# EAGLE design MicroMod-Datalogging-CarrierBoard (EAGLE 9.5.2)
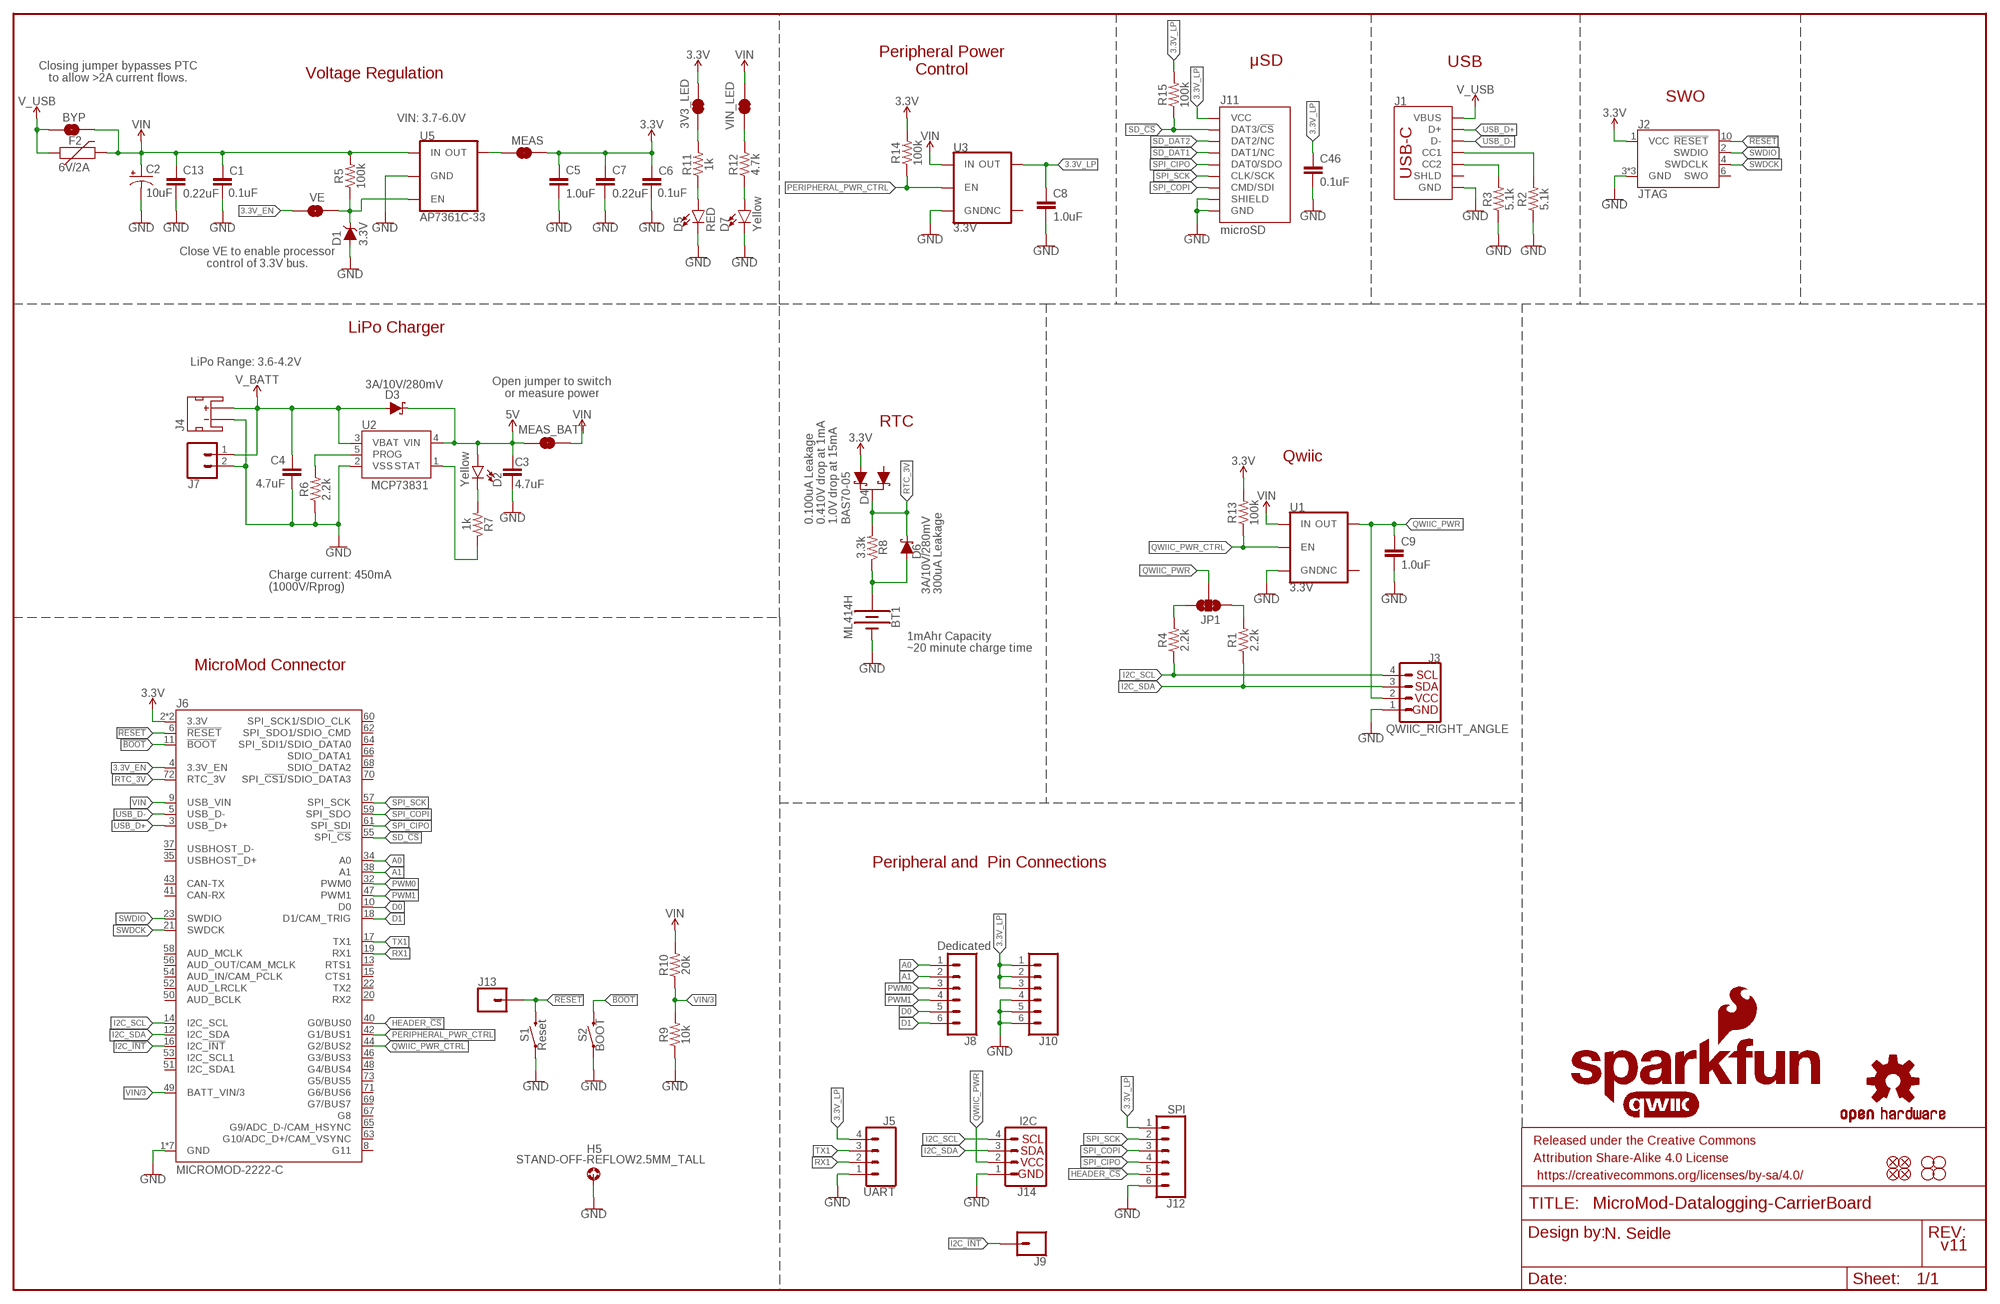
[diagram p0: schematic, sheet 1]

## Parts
3V3_LED  JUMPER-SMT_2_NC_TRACE_SILK  [SMT-JUMPER_2_NC_TRACE_SILK]
BT1  ML414H  ML414H_IV01E_BATTERY  [ML414H_IV01E]
BYP  JUMPER-SMT_2_NO_SILK  [SMT-JUMPER_2_NO_SILK]
C1  0.1uF  0.1UF-0603-25V-(+80/-20%)  [0603]
C2  10uF  10UF-POLAR-EIA3216-16V-10%(TANT)  [EIA3216]
C3  4.7uF  4.7UF-0603-35V-(20%)  [0603]
C4  4.7uF  4.7UF-0603-6.3V-(10%)  [0603]
C5  1.0uF  1.0UF-0603-16V-10%  [0603]
C6  0.1uF  0.1UF-0603-25V-(+80/-20%)  [0603]
C7  0.22uF  0.22UF-0603-25V-10%  [0603]
C8  1.0uF  1.0UF-0603-16V-10%  [0603]
C9  1.0uF  1.0UF-0603-16V-10%  [0603]
C13  0.22uF  0.22UF-0603-25V-10%  [0603]
C46  0.1uF  0.1UF-0603-25V-(+80/-20%)  [0603]
D1  3.3V  DIODE-ZENER-MM3Z3V3T1G  [SOD-323]
D2  Yellow  LED-YELLOW0603  [LED-0603]
D3  3A/10V/280mV  DIODE-SCHOTTKY-BAT60A  [SOD-323]
D4  BAS70-05  DIODE-SCHOTTKY-DUAL  [SOT23-3]
D5  RED  LED-RED0603  [LED-0603]
D6  3A/10V/280mV  DIODE-SCHOTTKY-BAT60A  [SOD-323]
D7  Yellow  LED-YELLOW0603  [LED-0603]
F2  6V/2A  PPTC_6V2A  [1210]
FD1  FIDUCIALUFIDUCIAL  [FIDUCIAL-MICRO]
FD2  FIDUCIALUFIDUCIAL  [FIDUCIAL-MICRO]
FD3  FIDUCIALUFIDUCIAL  [FIDUCIAL-MICRO]
FD4  FIDUCIALUFIDUCIAL  [FIDUCIAL-MICRO]
FRAME1  FRAME-LEDGER  [CREATIVE_COMMONS]
H1  STAND-OFF  [STAND-OFF]
H2  STAND-OFF  [STAND-OFF]
H3  STAND-OFF  [STAND-OFF]
H4  STAND-OFF  [STAND-OFF]
H5  STAND-OFF-REFLOW2.5MM_TALL  [STAND-OFF-REFLOW-M2.5]
J1  USB_C_2-LAYER_PADS  [USB-C-16P-2LAYER-PADS]
J2  JTAG  CORTEX_JTAG_DEBUG_MINIMUM_PTH  [2X5-PTH-1.27MM]
J3  QWIIC_RIGHT_ANGLE  QWIIC_CONNECTORJS-1MM  [JST04_1MM_RA]
J4  JST_2MM_MALE  [JST-2-SMD]
J5  UART  CONN_041X04_NO_SILK  [1X04_NO_SILK]
J6  MICROMOD-2222-C  [M.2-CONNECTOR-E]
J7  CONN_021X02_NO_SILK  [1X02_NO_SILK]
J8  Dedicated  CONN_06NO_SILK_NO_POP  [1X06_NO_SILK]
J9  CONN_01PTH_NO_SILK_YES_STOP  [1X01_NO_SILK]
J10  CONN_06NO_SILK_NO_POP  [1X06_NO_SILK]
J11  microSD  MICRO-SD-SDIOPUSH-PUSH  [MICRO-SD-SOCKET]
J12  SPI  CONN_06NO_SILK_NO_POP  [1X06_NO_SILK]
J13  CONN_01PTH_NO_SILK_YES_STOP  [1X01_NO_SILK]
J14  I2C  I2C_STANDARD_NO_SILK  [1X04_NO_SILK]
JP1  JUMPER-SMT_3_2-NC_TRACE_SILK  [SMT-JUMPER_3_2-NC_TRACE_SILK]
LOGO1  SFE_LOGO_NAME_FLAME.1_INCH  [SFE_LOGO_NAME_FLAME_.1]
LOGO2  QWIIC_LOGO_CONNECTOR  [QWIIC_5.5MM]
LOGO3  OSHW-LOGOMINI  [OSHW-LOGO-MINI]
MEAS  JUMPER-COMBO_2_NC_TRACE  [COMBO-JUMPER_2_NC_TRACE]
MEAS_BATT  JUMPER-COMBO_2_NC_TRACE  [COMBO-JUMPER_2_NC_TRACE]
R1  2.2k  2.2KOHM-0603-1/10W-1%  [0603]
R2  5.1k  5.1KOHM5.1KOHM-0603-1/10W-1%  [0603]
R3  5.1k  5.1KOHM5.1KOHM-0603-1/10W-1%  [0603]
R4  2.2k  2.2KOHM-0603-1/10W-1%  [0603]
R5  100k  100KOHM-0603-1/10W-1%  [0603]
R6  2.2k  2.2KOHM-0603-1/10W-1%  [0603]
R7  1k  1KOHM-0603-1/10W-1%  [0603]
R8  3.3k  3.3KOHM-0603-1/10W-1%  [0603]
R9  10k  10KOHM-0603-1/10W-1%  [0603]
R10  20k  20KOHM-0603-1/10W-1%  [0603]
R11  1k  1KOHM-0603-1/10W-1%  [0603]
R12  4.7k  4.7KOHM-0603-1/10W-1%  [0603]
R13  100k  100KOHM-0603-1/10W-1%  [0603]
R14  100k  100KOHM-0603-1/10W-1%  [0603]
R15  100k  100KOHM-0603-1/10W-1%  [0603]
S1  Reset  MOMENTARY-SWITCH-SPST-SMD-5.2-TALL-REDUNDANT  [TACTILE_SWITCH_SMD_5.2MM]
S2  BOOT  MOMENTARY-SWITCH-SPST-SMD-5.2-TALL-REDUNDANT  [TACTILE_SWITCH_SMD_5.2MM]
U1  3.3V  V_REG_AP2112K-3.3V  [SOT23-5]
U2  MCP73831  [SOT23-5]
U3  3.3V  V_REG_AP2112K-3.3V  [SOT23-5]
U5  AP7361C-33  AP7361C-33FGEUDFN-8  [UDFN-8]
VE  JUMPER-SMT_2_NO_SILK  [SMT-JUMPER_2_NO_SILK]
VIN_LED  JUMPER-SMT_2_NC_TRACE_SILK  [SMT-JUMPER_2_NC_TRACE_SILK]

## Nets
3.3V: 3V3_LED.2 C5.1 C6.1 C7.1 D4.2(A1) J2.1(VCC) J6.2(3.3V) J6.74(3.3V) MEAS.2 MEAS.4 R13.2 R14.2
3.3V_EN: J6.4(3.3V_EN) VE.1
3.3V_EN_VE: D1.C R5.1 U5.5(EN) VE.2
3.3V_LP: C8.1 C46.1 J5.4 J10.1 J10.2 J10.3 J11.VCC J12.1 R15.2 U3.5(OUT)
5V: C3.1 D2.A D3.C MEAS_BATT.1 MEAS_BATT.3 U2.4(VIN)
!BOOT!: J6.11(!BOOT!) S2.3 S2.4
!RESET!: J2.10(!RESET) J6.6(!RESET!) J13.1 S1.3 S1.4
A0: J6.34(A0) J8.1
A1: J6.38(A1) J8.2
CHG_LED: R7.1 U2.1(STAT)
D0: J6.10(D0) J8.5
D1: J6.18(D1/CAM_TRIG) J8.6
GND: BT1.- C1.2 C2.- C3.2 C4.2 C5.2 C6.2 C7.2 C8.2 C9.2 C13.2 C46.2 D1.A D5.C D7.C H5.1 J1.GND J1.GND2(GND) J2.3(GND) J2.5(GND) J2.9(GND) J3.1 J4.1(-) J5.1 J6.1(GND) J6.7(GND) J6.33(GND) J6.36(GND) J6.39(GND) J6.45(GND) J6.75(GND) J7.2 J10.4 J10.5 J10.6 J11.CD1(SHIELD) J11.GND J11.GND1(GND) J11.GND3(GND) J12.6 J14.1 R2.1 R3.1 R6.1 R9.1 S1.1 S1.2 S2.1 S2.2 U1.2(GND) U2.2(VSS) U3.2(GND) U5.4(GND) U5.EP(GND)
HEADER_!CS!: J6.40(G0/BUS0) J12.5
I2C_!INT!: J6.16(I2C_!INT!) J9.1
I2C_SCL: J3.4 J6.14(I2C_SCL) J14.4 R4.1
I2C_SDA: J3.3 J6.12(I2C_SDA) J14.3 R1.1
N$1: MEAS.1 MEAS.3 U5.1(OUT)
N$2: JP1.3 R4.2
N$3: JP1.1 R1.2
N$4: D2.C R7.2
N$5: D5.A R11.1
N$6: 3V3_LED.1 R11.2
N$7: R6.2 U2.5(PROG)
N$8: R12.2 VIN_LED.1
N$9: D7.A R12.1
N$10: J1.A5(CC1) R2.2
N$11: J1.B5(CC2) R3.2
N$14: BT1.+ D6.A R8.1
PERIPHERAL_PWR_CTRL: J6.42(G1/BUS1) R14.1 U3.3(EN)
PWM0: J6.32(PWM0) J8.3
PWM1: J6.47(PWM1) J8.4
QWIIC_PWR: C9.1 J3.2 J14.2 JP1.2 U1.5(OUT)
QWIIC_PWR_CTRL: J6.44(G2/BUS2) R13.1 U1.3(EN)
RTC_3V: D4.3(C) D6.C J6.72(RTC_3V) R8.2
RX1: J5.2 J6.19(RX1)
SD_!CS!: J6.55(SPI_!CS!) J11.CS/DAT3(DAT3/!CS!) R15.1
SD_DAT1: J11.DAT1(DAT1/NC)
SD_DAT2: J11.DAT2(DAT2/NC)
SPI_CIPO: J6.61(SPI_SDI) J11.DO/DAT0(DAT0/SDO) J12.4
SPI_COPI: J6.59(SPI_SDO) J11.DI/CMD(CMD/SDI) J12.3
SPI_SCK: J6.57(SPI_SCK) J11.SCLK(CLK/SCK) J12.2
SWDCK: J2.4(SWDCLK) J6.21(SWDCK)
SWDIO: J2.2(SWDIO) J6.23(SWDIO)
TX1: J5.3 J6.17(TX1)
USB_D+: J1.A6(D+) J1.B6(D+) J6.3(USB_D+)
USB_D-: J1.A7(D-) J1.B7(D-) J6.5(USB_D-)
V_BATT: C4.1 D3.A J4.2(+) J7.1 U2.3(VBAT)
V_USB: BYP.1 F2.1 J1.VBUS1(VBUS) J1.VBUS2(VBUS)
VIN: BYP.2 C1.1 C2.+ C13.1 F2.2 J6.9(USB_VIN) MEAS_BATT.2 MEAS_BATT.4 R5.2 R10.2 U1.1(IN) U3.1(IN) U5.8(IN) VIN_LED.2
VIN/3: J6.49(BATT_VIN/3) R9.2 R10.1
Unconnected: D4.1(A) J1.SHLD1(SHLD) J1.SHLD2(SHLD) J1.SHLD3(SHLD) J1.SHLD4(SHLD) J2.6(SWO) J4.NC1(PAD1) J4.NC2(PAD2) J6.8(G11) J6.13(RTS1) J6.15(CTS1) J6.20(RX2) J6.22(TX2) J6.35(USBHOST_D+) J6.37(USBHOST_D-) J6.41(CAN-RX) J6.43(CAN-TX) J6.46(G3/BUS3) J6.48(G4/BUS4) J6.50(AUD_BCLK) J6.51(I2C_SDA1) J6.52(AUD_LRCLK) J6.53(I2C_SCL1) J6.54(AUD_IN/CAM_PCLK) J6.56(AUD_OUT/CAM_MCLK) J6.58(AUD_MCLK) J6.60(SPI_SCK1/SDIO_CLK) J6.62(SPI_SDO1/SDIO_CMD) J6.63(G10/ADC_D+/CAM_VSYNC) J6.64(SPI_SDI1/SDIO_DATA0) J6.65(G9/ADC_D-/CAM_HSYNC) J6.66(SDIO_DATA1) J6.67(G8) J6.68(SDIO_DATA2) J6.69(G7/BUS7) J6.70(SPI_!CS1!/SDIO_DATA3) J6.71(G6/BUS6) J6.73(G5/BUS5) U1.4(NC) U3.4(NC)

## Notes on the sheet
- Peripheral Power
  Control
- μSD | USB
- Closing jumper bypasses PTC
  to allow >2A current flows.
- Voltage Regulation
- SWO
- VIN: 3.7-6.0V
- Close VE to enable processor
  control of 3.3V bus.
- LiPo Charger
- LiPo Range: 3.6-4.2V
- Open jumper to switch
  or measure power
- RTC
- Qwiic
- 0.100uA Leakage
  0.410V drop at 1mA
  1.0V drop at 15mA
- Charge current: 450mA
  (1000V/Rprog)
- 300uA Leakage
- 1mAhr Capacity
- ~20 minute charge time
- MicroMod Connector
- Peripheral and  Pin Connections
- N. Seidle
- v11

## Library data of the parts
3V3_LED VIN_LED = SparkFun-Jumpers:JUMPER-SMT_2_NC_TRACE: Normally closed trace jumper
BT1 = SparkFun-Batteries:ML414H_IV01E_BATTERY: SEIKO ML414H-IV01E Reflowable Lithium Battery; PROD_ID: BATT-14267
BYP VE = SparkFun-Jumpers:JUMPER-SMT_2_NO: Normally open jumper
C1 C6 C46 = SparkFun-Capacitors:0.1UF: 0.1µF ceramic capacitors; PROD_ID: CAP-00810
C2 = SparkFun-Capacitors:10UF-POLAR: 10.0µF polarized capacitors; PROD_ID: CAP-00811
C3 = SparkFun-Capacitors:4.7UF: 4.7µF ceramic capacitors; PROD_ID: CAP-14106
C4 = SparkFun-Capacitors:4.7UF: 4.7µF ceramic capacitors; PROD_ID: CAP-08280
C5 C8 C9 = SparkFun-Capacitors:1.0UF: 1µF ceramic capacitors; PROD_ID: CAP-00868
C7 C13 = SparkFun-Capacitors:0.22UF: 0.22µF ceramic capacitors; PROD_ID: CAP-07822
D1 = SparkFun-DiscreteSemi:DIODE-ZENER: Zener Diode; PROD_ID: DIO-11284
D2 D7 = SparkFun-LED:LED-YELLOW: Yellow SMD LED; PROD_ID: DIO-09003
D3 D6 = SparkFun-DiscreteSemi:DIODE-SCHOTTKY: Schottky diode; PROD_ID: DIO-14072
D4 = SparkFun-DiscreteSemi:DIODE-SCHOTTKY-DUAL: Diodes Incorporated - BAS70-05 Dual Schottky Diode Two Schottky Diodes in a single SOT-23 package. Low reverse current (100 nA) Vf: Datasheet referenced for footprint; PROD_ID: DIO-14829
D5 = SparkFun-LED:LED-RED: Red SMD LED; PROD_ID: DIO-00819
F2 = SparkFun-Fuses:PPTC: Resettable Fuse PPTC; PROD_ID: RES-14313
FD1-FD4 = SparkFun-Aesthetics:FIDUCIAL: Fiducial Alignment Points
FRAME1 = SparkFun-Aesthetics:FRAME-LEDGER: Schematic Frame - Ledger
H1-H4 = SparkFun-Hardware:STAND-OFF: Stand Off
H5 = SparkFun-Hardware:STAND-OFF-REFLOW: Stand Off Reflow Compatible; PROD_ID: HW-14899
J1 = SparkFun-Connectors:USB_C: USB Type C 16Pin Connector Super Speed pins not available on the 16-pin purely SMD connector so this part is best for USB 2.0 implementations. D1 and D2 are tied together enabling D+/- no matter which way the cable is plugged into the connector. The two channel configuration pins (CC1/2) are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; PROD_ID: CONN-14122
J2 = SparkFun-Connectors:CORTEX_JTAG_DEBUG_MINIMUM: Cortex Debug Connector - 10 pin Supports JTAG debug, Serial Wire debug, and Serial Wire Viewer. PTH and SMD connector options available. General Connector Information Products: PTH Connector -via Digi-Key SparkFun PSoc SparkFun T
J3 = SparkFun-Connectors:QWIIC_CONNECTOR: SparkFun I2C Standard Qwiic Connector An SMD 1mm pitch JST connector makes it easy and quick (get it? Qwiic?) to connect I2C devices to each other. The Qwiic system enables fast and solderless connection between popular platforms and various sensors and actuators. We carry 200mm, 100mm, 50mm, and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; PROD_ID: CONN-13694
J4 = SparkFun-Connectors:JST_2MM_MALE: JST 2MM MALE RA CONNECTOR Two pin, compact surface mount connector. Commonly used as a battery input connection point. We really like the solid locking feeling and high current rating on these small connectors. We use these all the time as battery connectors. Mates to single-cell LiPo batteries.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; PROD_ID: CONN-11443; SF_ID: PRT-08612
J5 = SparkFun-Connectors:CONN_04: Multi connection point. Often used as Generic Header-pin footprint for 0.1 inch spaced/style header connections On any of the 0.1 inch spaced packages, you can populate with these: Break Away Headers - Straight (PRT-00116) Break Away Male Headers - Right Angle (PRT-00553) Female Headers (PRT-00115)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; PROD_ID: CONN-09696
J6 = SparkFun-MicroMod:MICROMOD: MicroMod Connector Description: A card edge connector and mating PCB connector to allow various MicroMod Processor Boards to be coupled with various carrier boards of different capabilities. Based on the M.2 standard.; PROD_ID: CONN-14877
J7 = SparkFun-Connectors:CONN_02: Multi connection point. Often used as Generic Header-pin footprint for 0.1 inch spaced/style header connections
J8 J10 J12 = SparkFun-Connectors:CONN_06: Multi connection point. Often used as Generic Header-pin footprint for 0.1 inch spaced/style header connections On any of the 0.1 inch spaced packages, you can populate with these: Break Away Headers - Straight (PRT-00116) Break Away Male Headers - Right Angle (PRT-00553) Female Headers (PRT-00115)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
J9 J13 = SparkFun-Connectors:CONN_01: Single connection point. Often used as Generic Header-pin footprint for 0.1 inch spaced/style header connections
J11 = SparkFun-Connectors:MICRO-SD-SDIO: microSD Socket for Transflash Push-push type µSD socket. tDoc lines correctly indicate media card edge positions when inserting (unlocked, locked, depressed). NOTE: CD1 and CD2 are connected internally, and the default detect state of the socket is detect pin to ground. SparkFun Products: WAV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; PROD_ID: CONN-07820
J14 = SparkFun-Connectors:I2C_STANDARD: SparkFun I2C Standard Pinout Header SparkFun has standardized on a pinout for all I2C based sensor breakouts. This pinout allows I2C boards to be plugged directly into the headers on Arduino Uno compatible boards, and to be daisy chained easily. Example SparkFun Products: SparkFun Atmospheric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
JP1 = SparkFun-Jumpers:JUMPER-SMT_3_2-NC_TRACE: Normally closed trace jumper (2 of 2 connections) This jumper has a trace between all three pads so they are normally closed (NC). Use a razor knife to open the connection(s). For best results follow the IPC guidelines for cutting traces: Cutout at least 0.063 mm (0.005 in). Remove all loose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
LOGO1 = SparkFun-Aesthetics:SFE_LOGO_NAME_FLAME: SparkFun Font Logo w/ Flame
LOGO2 = SparkFun-Aesthetics:QWIIC_LOGO: Qwiic Logos for placement on schematic and PCB. The 5.5mm silk logo is best for placing next to Qwiic connector.
LOGO3 = SparkFun-Aesthetics:OSHW-LOGO: Open-Source Hardware (OSHW) Logo
MEAS MEAS_BATT = SparkFun-Jumpers:JUMPER-COMBO_2_NC_TRACE
R1 R4 R6 = SparkFun-Resistors:2.2KOHM: 2.2kΩ resistor; PROD_ID: RES-08272
R2 R3 = SparkFun-Resistors:5.1KOHM; PROD_ID: RES-12083
R5 R13-R15 = SparkFun-Resistors:100KOHM: 100kΩ resistor; PROD_ID: RES-07828
R7 R11 = SparkFun-Resistors:1KOHM: 1kΩ resistor; PROD_ID: RES-07856
R8 = SparkFun-Resistors:3.3KOHM: 3.3kΩ resistor; PROD_ID: RES-07851
R9 = SparkFun-Resistors:10KOHM: 10kΩ resistor; PROD_ID: RES-00824
R10 = SparkFun-Resistors:20KOHM: 20kΩ resistor; PROD_ID: RES-09383
R12 = SparkFun-Resistors:4.7KOHM: 4.7kΩ resistor; PROD_ID: RES-07857
S1 S2 = SparkFun-Switches:MOMENTARY-SWITCH-SPST: Momentary Switch (Pushbutton) - SPST; PROD_ID: SWCH-14139
U1 U3 = SparkFun-IC-Power:V_REG_AP2112: AP2112 - 600mA CMOS LDO Regulator w/ Enable The AP2112 is CMOS process low dropout linear regulator with enable function, the regulator delivers a guaranteed 600mA (min.) continuous load current. Features Output Voltage Accuracy: ±1.5% Output Current: 600mA (Min.) Foldback Short Current Protection: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; PROD_ID: VREG-12457
U2 = SparkFun-IC-Power:MCP73831: MCP73831T Li-Ion, Li-Pol Controller Miniature single cell, fully integrated Li-Ion, Li-polymer charge management controller Datasheet SparkFun Products: SparkFun ESP32 Thing SparkFun 9DoF Razor IMU M0; PROD_ID: IC-09995
U5 = SparkFun-IC-Power:AP7361C-33FGE: AP7361C 3.3V LDO Regulator; PROD_ID: VREG-14094

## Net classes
0 default: width 0 mm, drill 0 mm
1 power: width 0.762 mm

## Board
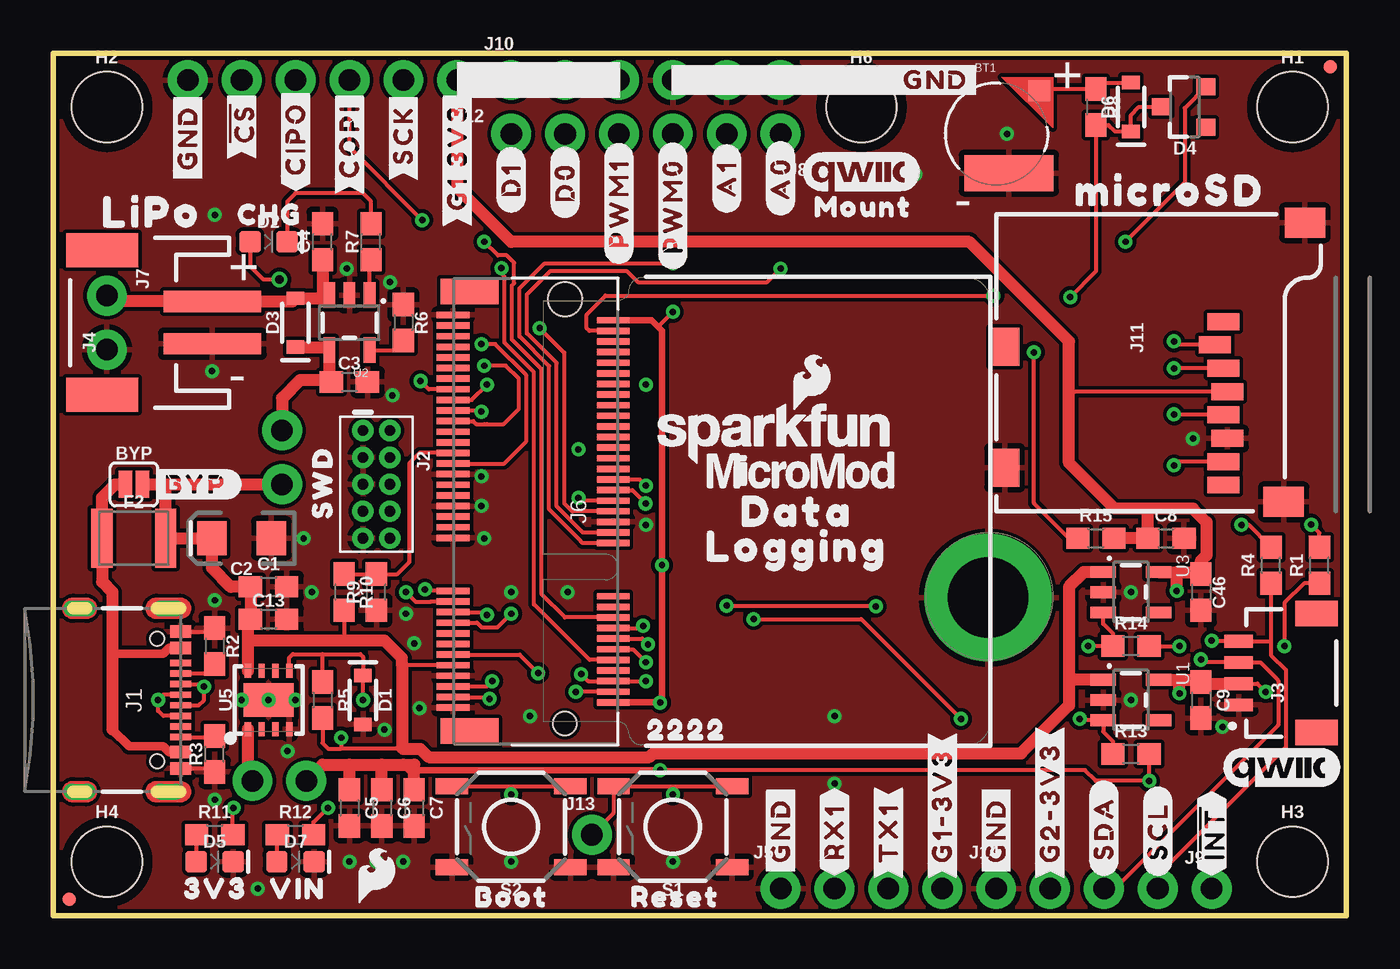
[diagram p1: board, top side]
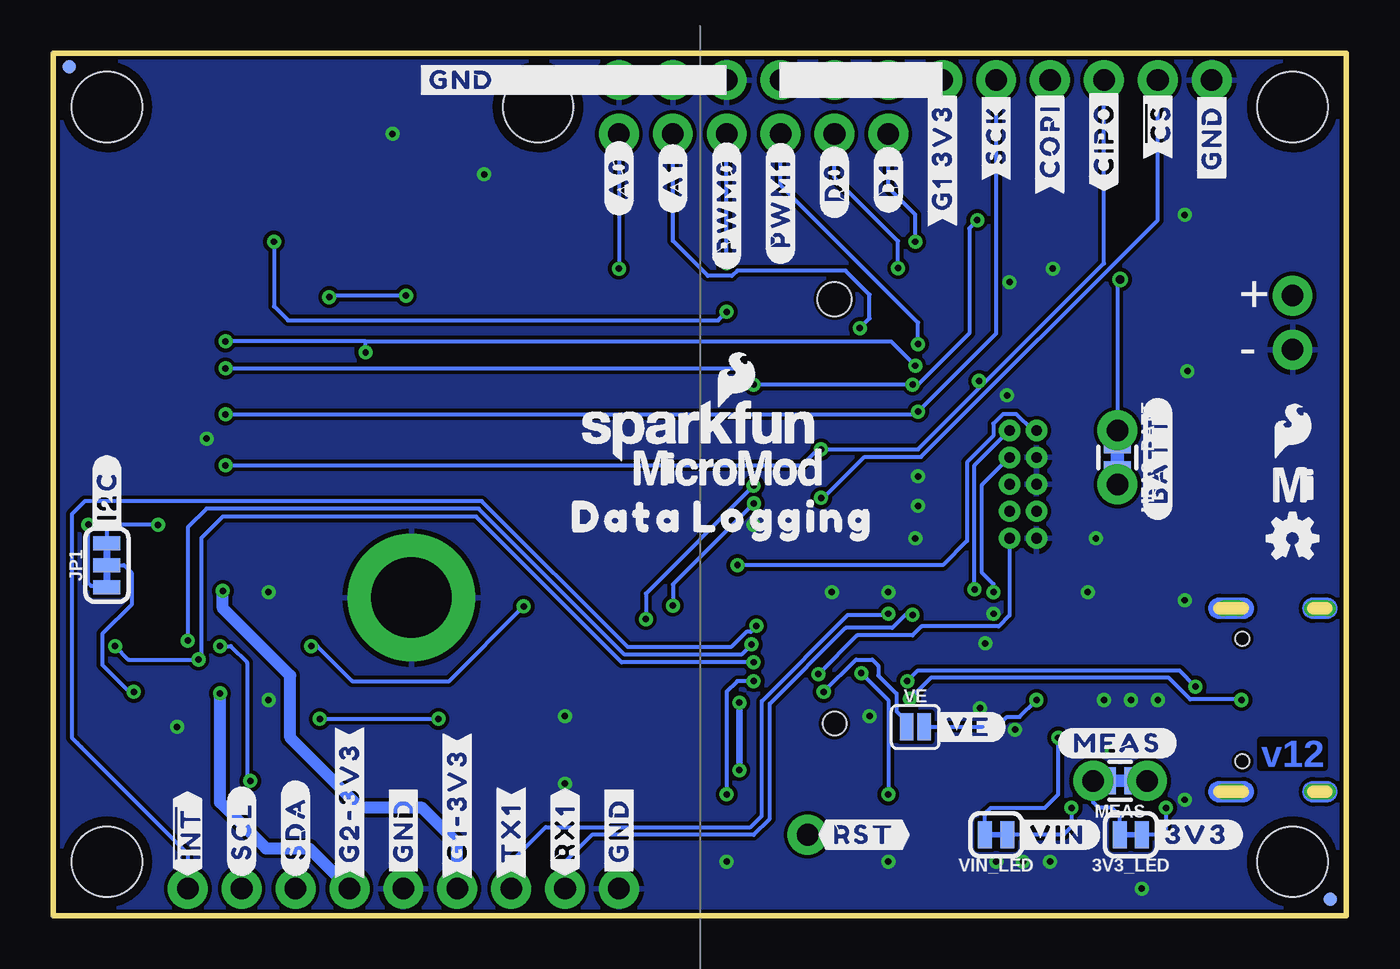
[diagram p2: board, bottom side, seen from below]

Size 60.96 x 40.64 mm. Coordinates in mm from the lower left corner, seen from the top.
Outline: 0,0 0,40.64 60.96,40.64 60.96,0 0,0
Copper layers (1*16): Top 0.035mm / dielectric 1.5mm / Bottom 0.035mm
Design rules "SparkFun-2-layer-TIGHT *": minimum track width 7mil, minimum drill 12mil, track to track 7mil, track to pad 7mil, pad to pad 7mil, via to via 7mil, smd to smd 7mil, copper to edge 7mil, drill to drill 7mil, minimum pad ring 7mil, minimum via ring 7mil, stop-mask expansion 4mil, vias tented up to drill 25mil, thermal gap 10mil

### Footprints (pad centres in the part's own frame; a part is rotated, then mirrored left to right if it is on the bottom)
SMT-JUMPER_2_NC_TRACE_SILK = smd 0.66 x 1.27: 1 -0.521,0; 2 0.521,0
ML414H_IV01E = smd 1 x 1: + 2.022,2.032 | smd 4.2 x 1.7: - 0.6,-1.85
SMT-JUMPER_2_NO_SILK = smd 0.635 x 1.27: 1 -0.406,0; 2 0.406,0
0603 = smd 1.1 x 1: 1 -0.85,0; 2 0.85,0
EIA3216 = smd 1.4 x 1.6: + 1.4,0; - -1.4,0
SOD-323 = smd 0.63 x 0.83: A 1.15,0; C -1.15,0
LED-0603 = smd 1 x 1: A -0.877,0; C 0.877,0
SOT23-3 = smd 0.8 x 0.9: 1 -0.95,-1; 2 0.95,-1; 3 0,1.1
1210 = smd 1 x 2.8: 1 -1.5,0; 2 1.5,0
FIDUCIAL-MICRO = smd 0.635 x 0.635: 1 0,0
STAND-OFF = hole 3.302: 0,0
STAND-OFF-REFLOW-M2.5 = drill 3.8 pad 6: 1 0,0
USB-C-16P-2LAYER-PADS = smd 0.3 x 1: A5 -1.25,-0.34; A6 -0.25,-0.34; A7 0.25,-0.34; A8 1.25,-0.34; B5 1.75,-0.34; B6 0.75,-0.34; B7 -0.75,-0.34; B8 -1.75,-0.34 | smd 0.6 x 1: GND -3.225,-0.34; GND2 3.225,-0.34; VBUS1 -2.45,-0.34; VBUS2 2.45,-0.34 | drill 0.4 pad 0.6 long: SHLD1 -4.318,-0.915; SHLD2 4.318,-0.915; SHLD3 -4.318,-5.095; SHLD4 4.318,-5.095 | hole 0.65: -2.89,-1.445; 2.89,-1.445
2X5-PTH-1.27MM = drill 0.508 pad 1: 1 -2.54,-0.635; 2 -2.54,0.635; 3 -1.27,-0.635; 4 -1.27,0.635; 5 0,-0.635; 6 0,0.635; 7 1.27,-0.635; 8 1.27,0.635; 9 2.54,-0.635; 10 2.54,0.635
JST04_1MM_RA = smd 0.6 x 1.35: 1 -1.5,0; 2 -0.5,0; 3 0.5,0; 4 1.5,0 | smd 1.2 x 2: NC1 2.8,-3.675; NC2 -2.8,-3.675
JST-2-SMD = smd 1 x 4.6: 1 -1,-3.7; 2 1,-3.7 | smd 1.6 x 3.4: NC1 -3.4,1.5; NC2 3.4,1.5
1X04_NO_SILK = drill 1.016 pad 1.88: 1 0,0; 2 2.54,0; 3 5.08,0; 4 7.62,0
M.2-CONNECTOR-E = smd 0.3 x 1.55: 1 9.25,-5.275; 2 9,2.275; 3 8.75,-5.275; 4 8.5,2.275; 5 8.25,-5.275; 6 8,2.275; 7 7.75,-5.275; 8 7.5,2.275; 9 7.25,-5.275; 10 7,2.275; 11 6.75,-5.275; 12 6.5,2.275; 13 6.25,-5.275; 14 6,2.275; 15 5.75,-5.275; 16 5.5,2.275; 17 5.25,-5.275; 18 5,2.275; 19 4.75,-5.275; 20 4.5,2.275; 21 4.25,-5.275; 22 4,2.275; 23 3.75,-5.275; 32 1.5,2.275; 33 1.25,-5.275; 34 1,2.275; 35 0.75,-5.275; 36 0.5,2.275; 37 0.25,-5.275; 38 0,2.275; 39 -0.25,-5.275; 40 -0.5,2.275; 41 -0.75,-5.275; 42 -1,2.275; 43 -1.25,-5.275; 44 -1.5,2.275; 45 -1.75,-5.275; 46 -2,2.275; 47 -2.25,-5.275; 48 -2.5,2.275; 49 -2.75,-5.275; 50 -3,2.275; 51 -3.25,-5.275; 52 -3.5,2.275; 53 -3.75,-5.275; 54 -4,2.275; 55 -4.25,-5.275; 56 -4.5,2.275; 57 -4.75,-5.275; 58 -5,2.275; 59 -5.25,-5.275; 60 -5.5,2.275; 61 -5.75,-5.275; 62 -6,2.275; 63 -6.25,-5.275; 64 -6.5,2.275; 65 -6.75,-5.275; 66 -7,2.275; 67 -7.25,-5.275; 68 -7.5,2.275; 69 -7.75,-5.275; 70 -8,2.275; 71 -8.25,-5.275; 72 -8.5,2.275; 73 -8.75,-5.275; 74 -9,2.275; 75 -9.25,-5.275 | smd 1.2 x 2.75: A1 10.35,-4.5; A2 -10.35,-4.5 | hole 1.1: 10,0 | hole 1.6: -10,0
1X02_NO_SILK = drill 1.016 pad 1.88: 1 0,0; 2 2.54,0
1X06_NO_SILK = drill 1.016 pad 1.88: 1 0,0; 2 2.54,0; 3 5.08,0; 4 7.62,0; 5 10.16,0; 6 12.7,0
1X01_NO_SILK = drill 1.016 pad 1.88: 1 0,0
MICRO-SD-SOCKET = smd 1.8 x 1.4: CD1 -2.05,0.4; CD2 -7.75,0.4 | smd 0.8 x 1.5: CS/DAT3 -7.84,10.3; DAT1 -1.24,10.7; DAT2 -8.94,10.7; DI/CMD -6.74,10.7; DO/DAT0 -2.34,10.7; GND -3.44,10.9; SCLK -4.54,10.7; VCC -5.64,10.9 | smd 1.4 x 1.9: GND1 -13.6,14.55; GND3 -0.45,13.55
SMT-JUMPER_3_2-NC_TRACE_SILK = smd 0.66 x 1.27: 1 -1.041,0; 2 0,0; 3 1.041,0
COMBO-JUMPER_2_NC_TRACE = smd 0.635 x 1.27: 1 -0.508,0; 2 0.508,0 | drill 1.016 pad 1.88: 3 -1.27,0; 4 1.27,0
TACTILE_SWITCH_SMD_5.2MM = smd 1.524 x 0.762: 1 -2.794,1.905; 2 2.794,1.905; 3 -2.794,-1.905; 4 2.794,-1.905
SOT23-5 = smd 0.55 x 1.2: 1 -0.95,-1.3; 2 0,-1.3; 3 0.95,-1.3; 4 0.95,1.3; 5 -0.95,1.3
UDFN-8 = smd 0.3 x 0.65: 1 -0.975,-1.375; 2 -0.325,-1.375; 3 0.325,-1.375; 4 0.975,-1.375; 5 0.975,1.375; 6 0.325,1.375; 7 -0.325,1.375; 8 -0.975,1.375 | smd 2.35 x 1.6: EP 0,0

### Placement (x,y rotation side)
3V3_LED  10.16,3.81 180 bottom
BT1  44.45,36.83 0 top
BYP  3.81,20.32 0 top
C1  10.16,15.49 0 top
C2  8.89,17.78 180 top
C3  13.97,25.15 0 top
C4  12.7,31.75 90 top
C5  13.97,5.08 270 top
C6  15.49,5.08 270 top
C7  17.02,5.08 270 top
C8  52.45,17.78 0 top
C9  54.1,10.16 270 top
C13  10.16,13.97 0 top
C46  54.1,15.24 270 top
D1  14.61,10.16 270 top
D2  10.16,31.75 0 top
D3  11.43,27.94 90 top
D4  53.34,38.1 90 top
D5  7.62,2.54 0 top
D6  50.8,38.1 90 top
D7  11.43,2.54 0 top
F2  3.81,17.78 0 top
FD1  0.76,0.76 0 top
FD2  60.2,40.01 0 top
FD3  0.76,0.76 0 bottom
FD4  60.2,40.01 0 bottom
FRAME1  not placed on the board
H1  58.42,38.1 0 top
H2  2.54,38.1 0 top
H3  58.42,2.54 0 top
H4  2.54,2.54 0 top
H5  44.07,14.99 0 top
H6  STAND-OFF  [STAND-OFF]  38.1,38.1 0 top
J1  6.35,10.16 270 top
J2  15.24,20.32 270 top
J3  55.88,11.43 90 top
J4  3.81,27.94 90 top
J5  34.29,1.27 0 top
J6  24.13,19.05 270 top
J7  2.54,29.21 270 top
J8  34.29,36.83 180 top
J9  54.61,1.27 0 top
J10  21.59,39.37 0 top
J11  44.45,19.05 270 top
J12  19.05,39.37 180 top
J13  25.4,3.81 0 top
J14  44.45,1.27 0 top
JP1  58.42,16.51 90 bottom
LOGO1  34.04,22.73 0 top
LOGO2  57.91,6.99 0 top
LOGO3  2.54,17.78 0 bottom
LOGO4  SFE_LOGO_NAME_FLAME.1_INCH  [SFE_LOGO_NAME_FLAME_.1]  30.48,22.86 0 bottom
LOGO5  QWIIC_LOGO_CONNECTOR  [QWIIC_5.5MM]  38.1,35.05 0 top
MEAS  10.67,6.35 180 bottom
MEAS_BATT  10.79,21.59 270 bottom
R1  59.69,16.51 90 top
R2  7.62,12.7 270 top
R3  7.62,7.62 90 top
R4  57.4,16.51 90 top
R5  12.7,10.16 270 top
R6  16.51,27.94 270 top
R7  14.99,31.75 90 top
R8  49.15,38.1 270 top
R9  15.24,15.24 90 top
R10  13.72,15.24 270 top
R11  7.62,3.81 0 top
R12  11.43,3.81 0 top
R13  50.8,7.62 0 top
R14  50.8,12.7 0 top
R15  49.15,17.78 0 top
S1  29.21,4.19 180 top
S2  21.59,4.19 180 top
U1  50.8,10.16 270 top
U2  13.97,27.94 180 top
U3  50.8,15.24 270 top
U5  10.16,10.16 0 top
U$1  [SFE_LOGO_FLAME_.1]  2.54,22.86 0 bottom
U$2  [#D1#0]  21.59,33.15 90 bottom
U$3  [#D0#0]  24.13,32.89 90 bottom
U$4  [#3V3#2]  9.27,3.81 0 bottom
U$5  [#BATT#0]  8.89,18.67 90 bottom
U$6  [#GND#0]  6.35,34.42 90 top
U$7  [#SCK#0]  16.51,34.67 90 top
U$8  [#SCK#0]  16.51,34.67 90 bottom
U$9  [#PWM1#1]  26.67,30.73 90 bottom
U$10  [#PWM0#0]  29.21,30.48 90 bottom
U$11  [MICROSD0]  47.12,34.16 0 top
U$12  [#A1#2]  31.75,33.15 90 bottom
U$13  [#A0#3]  34.29,33.02 90 bottom
U$14  [MOUNT0]  35.18,33.4 0 top
U$15  [LIPO0]  1.27,33.15 0 top
U$16  [DATA0]  31.37,19.05 0 top
U$17  [#RX1#1]  36.83,1.91 90 bottom
U$18  [#GND#0]  6.35,34.42 90 bottom
U$19  [LOGGING1]  29.72,17.4 0 top
U$20  [22220]  27.3,8.76 0 top
U$21  [#TX1#2]  39.37,1.78 90 bottom
U$22  [#I2C#0]  58.42,17.91 90 bottom
U$23  [DATA0]  37.59,18.8 0 bottom
U$24  [#GND#0]  34.29,1.78 90 top
U$25  [#G1#3V3#0]  41.91,1.78 90 bottom
U$26  [LOGGING1]  31.88,18.8 0 bottom
U$27  [#GND#0]  34.29,1.78 90 bottom
U$28  [#MEAS#3]  13.59,8.13 0 bottom
U$29  [#G2#3V3#3]  46.99,1.78 90 bottom
U$30  [#RST#0]  24.89,3.81 0 bottom
U$31  [#SDA#4]  49.53,1.91 90 bottom
U$32  [#GND#0]  44.45,1.78 90 top
U$33  [#VIN#1]  15.62,3.81 0 bottom
U$34  [#GND#0]  43.94,39.37 0 bottom
U$35  [#SCL#5]  52.07,1.91 90 bottom
U$36  [#GND#0]  44.45,1.78 90 bottom
U$37  [MICROMOD_LOGO_.35]  29.21,21.08 0 bottom
U$38  [##INT##6]  54.61,1.91 90 bottom
U$39  [#CIPO#0]  11.43,34.16 90 top
U$40  [#CIPO#0]  11.43,34.16 90 bottom
U$41  [#VE#0]  19.56,8.89 0 bottom
U$42  [#GND#0]  39.37,39.37 0 top
U$50  [##CS##0]  8.89,35.69 90 top
U$51  [##CS##0]  8.89,35.69 90 bottom
U$62  [MICROMOD_MI_LOGO_.35]  2.54,20.32 0 bottom
U$63  [MICROMOD_LOGO_.35]  35.18,20.95 0 top
U$64  [#G1_3V3#0]  19.05,32.51 90 top
U$65  [#G1_3V3#0]  19.05,32.51 90 bottom
U$66  [SFE_LOGO_FLAME_.1]  15.24,1.91 0 top
U$72  [#COPI#0]  13.97,34.04 90 top
U$73  [#COPI#0]  13.97,34.04 90 bottom
U$76  [#D1#0]  21.59,33.15 90 top
U$77  [#D0#0]  24.13,32.89 90 top
U$78  [#A0#3]  34.29,33.02 90 top
U$79  [#A1#2]  31.75,33.15 90 top
U$80  [#PWM0#0]  29.21,30.48 90 top
U$81  [#PWM1#1]  26.67,30.73 90 top
U$82  [##INT##6]  54.61,1.91 90 top
U$83  [#G2#3V3#3]  46.99,1.78 90 top
U$86  [#RX1#1]  36.83,1.91 90 top
U$87  [#SCL#5]  52.07,1.91 90 top
U$88  [#SDA#4]  49.53,1.91 90 top
U$89  [#TX1#2]  39.37,1.78 90 top
U$90  [#G1#3V3#0]  41.91,1.78 90 top
U$91  [BOOT0]  19.18,0.89 0 top
U$92  [RESET1]  26.54,0.89 0 top
U$93  [3V30]  5.46,1.27 0 top
U$94  [VIN1]  9.53,1.27 0 top
U$95  [#BYP#3]  4.57,20.32 0 top
U$96  [CHG1]  8,33.02 0 top
U$97  [SWD0]  12.7,18.03 90 top
VE  20.32,8.89 0 bottom
VIN_LED  16.51,3.81 180 bottom

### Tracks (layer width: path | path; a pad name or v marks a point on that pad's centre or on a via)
3.3V  (via drill 0.3)
  Top 0.178: v29.21,28.45 28.51,27.75 | D4.2 53.34,38.05 53.34,34.54 v50.55,31.75 | 28.7,6.86 48.64,6.86 49.15,6.35 v51.66,6.35 51.69,6.35 51.65,6.39 R13.2 | R14.2 v53.09,12.7
  Top 0.305: 28.7,25.4 28.7,27.56 28.51,27.75 28.21,28.05 J6.74 | 28.7,25.4 v28.7,16.51 28.7,10.03 | 28.7,10.03 28.68,10.05 28.61,10.05 | J6.2 28.61,10.05 | 28.7,6.86 v28.61,6.86 16.76,6.86 16.51,7.11 | 28.7,10.03 28.63,10.03 | 28.63,10.03 28.61,10.05 | 28.63,10.03 v28.61,10.03 | 28.7,25.4
  Top 0.559: 13.97,7.11 12.7,7.11 MEAS.4 | 13.97,7.11 15.49,7.11 | 15.49,7.11 16.51,7.11 17.02,7.11 C7.1 | C5.1 13.97,7.11 | C6.1 15.49,7.11
  Bottom 0.178: MEAS.2 MEAS.4 11.94,5.33 11.68,5.08 11.05,5.08 10.68,4.71 3V3_LED.2 | v50.55,31.75 50.55,28.7 49.89,28.04 29.62,28.04 v29.21,28.45 | J2.1 14.79,22.86 15.56,23.63 16.19,23.63 16.64,23.18 16.64,22.6 17.88,21.36 17.88,17.65 19.02,16.51 v28.7,16.51 | v53.09,12.7 52.58,12.7 51.82,11.94 51.82,6.5 v51.66,6.35
  Bottom 0.305: v28.61,10.03 v28.61,6.86
3.3V_EN  (via drill 0.3)
  Top 0.178: J6.4 v24.64,10.54
  Bottom 0.178: v24.64,10.54 23.11,12.06 22.35,12.06 22.06,11.77 22.06,11.31 21.21,10.46 21.21,9.63 20.73,9.14 VE.1
3.3V_EN_VE  (via drill 0.3)
  Top 0.178: v14.61,10.16 D1.C 14.61,12.19 14.48,12.32 12.7,12.32 | U5.5 11.13,12.15 11.3,12.32 12.7,12.32 | R5.1 12.7,12.32
  Bottom 0.178: VE.2 16.46,8.89 15.99,9.36 15.4,9.36 v14.61,10.16
3.3V_LP  (via drill 0.3)
  Top 0.178: J11.VCC 47.93,24.69 47.88,24.64
  Top 0.559: J10.3 J10.2 J10.1 J12.1 19.05,34.29 21.59,31.75 43.18,31.75 47.88,27.05 47.88,24.64 47.88,21.34 50.04,19.18 51.56,19.18 | 51.56,19.18 53.72,19.18 54.36,18.54 54.36,16.98 54.1,16.73 C46.1 54,16.19 52.96,16.19 | U3.5 52.96,16.19 | v52.96,15.3 52.96,16.19 | R15.2 C8.1 51.6,19.14 51.56,19.18
  Bottom 0.559: J5.4 41.91,3.43 43.56,5.08 46.48,5.08 49.78,8.38 49.78,11.3 52.96,14.48 v52.96,15.3
5V  (via drill 0.38)
  Top 0.178: D2.A 9.28,30.59 9.91,29.97 v10.67,29.97
  Top 0.559: D3.C 12.87,26.79 U2.4 13.02,25.25 | 13.02,25.25 C3.1 | 13.02,25.25 11.66,25.25 10.79,24.38 MEAS_BATT.3
  Bottom 0.178: MEAS_BATT.1 MEAS_BATT.3 10.79,29.84 v10.67,29.97
!BOOT!  (via drill 0.3)
  Top 0.178: v22.86,11.43 21.99,12.3 J6.11 | S2.4 21.59,6.1 | 21.59,6.1 S2.3 | v21.59,5.71 21.59,6.1
  Bottom 0.178: v22.86,11.43 21.59,10.16 v21.59,5.71
!RESET!  (via drill 0.3)
  Top 0.178: v27.94,11.05 J6.6 25.22,11.05 v24.89,11.38 | 29.21,6.1 S1.4 26.42,4.83 J13.1 | 29.21,6.1 S1.3 | v29.21,5.71 29.21,6.1
  Bottom 0.178: J2.10 15.88,14.14 16.39,13.63 20.03,13.63 20.45,13.21 23.06,13.21 v24.89,11.38 | v27.94,11.05 28.7,11.05 29.21,10.54 v29.21,5.71
A0  (via drill 0.3)
  Top 0.178: v34.29,30.48 33.66,29.84 27.56,29.84 27.03,30.38 23.44,30.38 22.34,29.27 22.34,27.44 23.73,26.04 23.73,19.28 24.97,18.05 J6.34
  Bottom 0.178: J8.1 v34.29,30.48
A1  (via drill 0.3)
  Top 0.178: v22.93,27.69 24.09,26.53 24.09,19.43 24.47,19.05 J6.38
  Bottom 0.178: J8.2 31.75,31.8 30.09,30.14 28.96,30.14 28.71,30.39 23.61,30.39 22.48,29.26 22.48,28.14 v22.93,27.69
CHG_LED
  Top 0.178: U2.1 14.92,30.83 R7.1
D0  (via drill 0.3)
  Top 0.178: v21.13,30.51 21.13,30.25 21.27,30.11 21.27,27 22.67,25.6 22.67,14.67 25.29,12.05 J6.10
  Bottom 0.178: v21.13,30.51 21.13,31.78 24.13,34.77 J8.5
D1  (via drill 0.3)
  Top 0.178: v20.32,31.75 20.96,31.11 21.38,31.11 21.73,30.75 21.73,29.8 21.63,29.7 21.63,27.14 23.02,25.75 23.02,15.15 24.13,14.05 J6.18
  Bottom 0.178: v20.32,31.75 20.32,33.02 21.59,34.29 J8.6
GND  (via drill 0.3)
  Top 0.178: J1.GND 7.46,13.38 R2.1 | J1.GND2 7.46,6.93 R3.1
  other vias: 7.62,5.46 11.05,7.75 10.16,10.16 11.43,10.16 8.89,10.16 15.62,8.76 17.27,9.78 13.97,2.54 15.24,2.54 16.51,2.54 16.64,14.22 12.19,15.24 11.81,17.78 7.62,14.86 15.88,29.84 7.49,25.65 7.62,33.02 27.94,18.41 20.19,19.3 20.19,20.7 20.32,17.78 55.12,8.89 53.72,22.48 40.64,34.92 24.26,15.24 21.59,15.24 36.83,9.4 36.83,6.22 29.21,2.54 21.59,2.54 9.65,1.27 44.96,36.83 17.02,12.83 22.48,9.4 13.84,30.48 16,24.51 50.8,15.24 50.8,10.16
  pour Bottom (isolate 0.178): 0,40.64 60.96,40.64 60.96,0 0,0
  pour Top (isolate 0.178): 0,40.64 60.96,40.64 60.96,0 0,0
HEADER_!CS!  (via drill 0.3)
  Top 0.178: J6.40 24.9,19.55 v24.77,19.68
  Bottom 0.178: J12.5 8.89,32.77 20.05,21.61 22.71,21.61 24.64,19.68 v24.77,19.68
I2C_!INT!  (via drill 0.3)
  Top 0.178: J6.16 27.72,13.55 v27.81,13.65
  Bottom 0.178: v27.81,13.65 28.09,13.37 28.29,13.37 29.01,12.65 33.87,12.65 40.75,19.53 58.42,19.53 58.7,19.53 59.46,19.53 60.07,18.92 60.07,8.38 59.82,8.13 59.63,7.94 54.61,2.92 J9.1
I2C_SCL  (via drill 0.3)
  Top 0.178: J14.4 52.07,1.91 58.1,7.94 58.1,11.58 57.4,12.27 57.4,12.95 | J6.14 27.77,13.05 v28.04,12.78 | R4.1 57.4,12.95 | v54.61,12.95 54.63,12.93 J3.4 57.38,12.93 57.4,12.95
  Bottom 0.178: v28.04,12.78 28.52,12.29 34.02,12.29 40.9,19.18 53.72,19.18 54.61,18.29 v54.61,12.95
I2C_SDA  (via drill 0.3)
  Top 0.178: J14.3 50.04,1.27 57.75,8.98 57.75,11.09 56.9,11.93 J3.3 54.24,11.93 v54.1,12.07 | J6.12 27.33,12.55 v27.94,11.94 | v58.04,12.7 58.04,14.73 58.97,15.66 R1.1
  Bottom 0.178: v27.94,11.94 34.16,11.94 41.02,18.8 52.96,18.8 53.98,17.78 53.98,12.2 v54.1,12.07 57.41,12.07 v58.04,12.7
N$1
  Top 0.559: U5.1 9.19,6.56 MEAS.3
  Bottom 0.178: MEAS.3 MEAS.1
N$2  (via drill 0.3)
  Top 0.178: R4.2 56.35,18.41 v56.01,18.41
  Bottom 0.178: v56.01,18.41 58.17,18.41 58.42,18.16 JP1.3
N$3  (via drill 0.3)
  Top 0.178: R1.2 59.69,18.03 v59.3,18.43
  Bottom 0.178: v59.3,18.43 59.3,18.02 59.32,17.99 59.32,15.69 59.16,15.53 58.48,15.53 JP1.1
N$4
  Top 0.178: R7.2 14.99,33.66 14.61,34.04 11.43,34.04 11.04,33.64 D2.C
N$5
  Top 0.178: R11.1 6.74,3.78 D5.A
N$6  (via drill 0.3)
  Top 0.178: R11.2 8.47,5.04 v8.51,5.08
  Bottom 0.178: v8.51,5.08 8.51,4.06 8.76,3.81 3V3_LED.1
N$7
  Top 0.178: U2.5 16.06,26.64 R6.2
N$8  (via drill 0.3)
  Top 0.178: R12.2 12.28,4.41 v12.95,5.08
  Bottom 0.178: v12.95,5.08 12.95,4.19 13.34,3.81 VIN_LED.1
N$9
  Top 0.178: R12.1 10.55,3.78 D7.A
N$10
  Top 0.178: J1.A5 7.18,11.41 R2.2
N$11
  Top 0.178: J1.B5 7.56,8.41 R3.2
N$14
  Top 0.178: BT1.+ 46.56,38.95 R8.1 49.45,39.25 D6.A
PERIPHERAL_PWR_CTRL  (via drill 0.3)
  Top 0.178: J6.42 27.3,20.05 v27.93,19.42 | v38.77,14.57 31.79,14.57 v31.75,14.61 | U3.3 49.5,13.75 49.95,13.3 R14.1 v48.79,12.7
  Bottom 0.178: v27.93,19.42 31.75,15.6 v31.75,14.61 | v48.79,12.7 48.5,12.7 46.85,11.05 42.29,11.05 v38.77,14.57
PWM0  (via drill 0.3)
  Top 0.178: v29.21,30.73 23.17,30.73 21.98,29.55 21.98,27.29 23.38,25.89 23.38,19.14 24.88,17.64 24.88,17.63 24.97,17.55 J6.32
  Bottom 0.178: v29.21,30.73 J8.3
PWM1  (via drill 0.3)
  Top 0.178: v20.19,26.92 20.84,26.92 22.31,25.45 22.31,22.35 21.26,21.3 J6.47
  Bottom 0.178: v20.19,26.92 20.19,27.94 26.67,34.42 J8.4
QWIIC_PWR  (via drill 0.3)
  Top 0.178: J3.2 56.76,10.93 v57.15,10.54
  Top 0.559: J3.2 54.18,10.93 C9.1 54,11.11 53.09,11.11 | U1.5 53.09,11.11 | v53.09,10.47 53.09,11.11
  Bottom 0.178: JP1.2 57.61,16.51 57.26,16.16 57.26,14.65 58.64,13.28 58.64,11.82 57.36,10.54 v57.15,10.54
  Bottom 0.559: J14.2 48.9,3.17 50.93,3.17 53.09,5.33 v53.09,10.47
QWIIC_PWR_CTRL  (via drill 0.3)
  Top 0.178: J6.44 27.65,20.55 v27.94,20.26 | v33.02,13.97 38.1,13.97 v42.8,9.27 | R13.1 49.95,8.22 49.5,8.67 U1.3 48.45,9.21 v48.39,9.27
  Bottom 0.178: v27.94,20.26 33.02,15.18 v33.02,13.97 | v48.39,9.27 v42.8,9.27
RTC_3V  (via drill 0.3)
  Top 0.178: v44.32,29.21 26.04,29.21 25.15,28.32 25.15,27.69 25.28,27.55 J6.72 | v47.94,29.15 49.15,30.35 R8.2 49.74,37.25 50.05,36.95 D6.C 50.8,37.72 51.18,38.1 D4.3
  Bottom 0.178: v44.32,29.21 47.88,29.21 v47.94,29.15
RX1  (via drill 0.3)
  Top 0.178: v20.45,14.17 20.32,14.3 J6.19
  Bottom 0.178: v20.45,14.17 20.8,14.17 21.41,13.56 23.6,13.56 27.18,9.99 27.18,4.57 27.94,3.81 35.56,3.81 36.83,2.54 J5.2
SD_!CS!  (via drill 0.3)
  Top 0.178: J11.CS/DAT3 52.99,26.89 v52.83,27.05 | R15.1 47.88,17.78 46.23,19.43 v46.23,26.54 | J6.55 19.8,23.3 19.95,23.15 20.32,23.15 20.44,23.15 21.23,23.15 21.96,23.88 21.96,25.29 21.34,25.91 v20.32,25.91
  Bottom 0.178: 46.23,27.05 v52.83,27.05 | v46.23,26.54 46.23,27.05 | v20.32,25.91 21.46,27.05 46.23,27.05
SPI_CIPO  (via drill 0.3)
  Top 0.178: J11.DO/DAT0 53.01,21.39 v52.83,21.21 | J6.61 17.7,24.8 v17.32,25.19
  Bottom 0.178: J12.4 11.43,30.73 16.97,25.19 | v52.83,21.21 25.65,21.21 24.83,22.04 v24.77,21.97 20.19,21.97 16.97,25.19 | v17.32,25.19 16.97,25.19
SPI_COPI  (via drill 0.3)
  Top 0.178: J11.DI/CMD 52.84,25.79 v52.83,25.78 | J12.3 13.97,36.2 v17.4,32.77 | J6.59 19.73,24.3 v20.45,25.02
  Bottom 0.178: v52.83,25.78 29.21,25.78 28.7,25.78 v27.94,25.02 v20.45,25.02 20.19,25.02 17.78,27.43 17.78,32.38 v17.4,32.77
SPI_SCK  (via drill 0.3)
  Top 0.178: J11.SCLK 52.86,23.59 v52.83,23.62 | J6.57 20.14,23.8 v20.19,23.75
  Bottom 0.178: J12.2 16.51,27.43 v20.19,23.75 20.32,23.62 v52.83,23.62
SWDCK  (via drill 0.3)
  Top 0.178: J6.21 17.8,14.8 17.77,14.77 17.11,14.77 v16.64,15.24
  Bottom 0.178: v16.64,15.24 16.64,15.62 17.17,16.15 17.17,20.3 J2.4
SWDIO  (via drill 0.3)
  Top 0.178: J6.23 17.59,15.3 v17.53,15.37
  Bottom 0.178: v17.53,15.37 17.53,21.21 J2.2
TX1  (via drill 0.3)
  Top 0.178: v21.59,14.22 20.94,13.58 20.2,13.58 19.98,13.8 J6.17
  Bottom 0.178: v21.59,14.22 21.64,14.17 23.5,14.17 27.56,10.11 27.56,4.7 28.09,4.17 37.74,4.17 39.37,2.54 J5.3
USB_D+  (via drill 0.3)
  Top 0.178: J1.A6 5.2,10.41 v4.95,10.16 4.95,9.65 5.2,9.41 J1.B6 | v20.57,10.21 20.48,10.3 J6.3
  Bottom 0.178: v4.95,10.16 4.99,10.2 7.36,10.2 8.36,11.2 19.59,11.2 v20.57,10.21
USB_D-  (via drill 0.3)
  Top 0.178: J1.B7 6.99,10.91 v7.11,10.79 7.11,10.16 6.86,9.91 J1.A7 | v20.7,11.05 20.45,10.8 J6.5
  Bottom 0.178: v20.7,11.05 20.2,11.55 7.87,11.55 v7.11,10.79
V_BATT
  Top 0.559: J7.1 2.81,28.94 J4.2 11.28,28.94 D3.A 12.57,29.09 | 12.57,29.09 12.87,29.09 U2.3 | C4.1 12.7,29.22 12.57,29.09
V_USB
  Top 0.406: J1.VBUS2 5.46,7.71 5.2,7.98 3.58,7.98 2.79,8.76 | J1.VBUS1 5.46,12.61 5.2,12.34 2.95,12.34 2.79,12.19
  Top 0.559: BYP.1 2.92,20.32 2.31,19.71 F2.1 2.31,15.72 2.79,15.24 2.79,12.19 2.79,8.76
VIN  (via drill 0.3)
  Top 0.178: R10.2 13.72,12.95 | R5.2 12.7,8.13 12.95,7.87 13.59,7.87 | 16.45,11.81 16.46,11.8 J6.9 | v13.59,8.38 13.59,7.87 | 16.45,7.91 16.41,7.87 13.59,7.87
  Top 0.559: BYP.2 5.33,20.32 | 5.33,20.32 5.31,20.3 F2.2 C2.+ 7.49,16.39 8.38,15.49 C1.1 C13.1 9.19,13.85 9.19,12.95 | U5.8 9.19,12.95 | 9.19,12.95 13.72,12.95 15.62,12.95 16.45,12.13 16.45,11.81 16.45,7.91 16.51,7.85 17.32,7.85 17.7,7.47 28.11,7.47 28.29,7.64 45.62,7.64 47.88,9.91 47.88,11.05 | 5.33,20.32 MEAS_BATT.4 | U3.1 48.58,16.19 47.88,15.49 47.88,11.05 | U1.1 47.94,11.11 47.88,11.05
  Bottom 0.178: MEAS_BATT.2 MEAS_BATT.4 | VIN_LED.2 17.03,4.81 16.76,5.08 14.22,5.08 13.59,5.71 v13.59,8.38
VIN/3
  Top 0.178: R10.1 R9.2 16.22,16.09 16.79,16.66 16.79,21.31 17.27,21.8 J6.49

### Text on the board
Bottom: v12
tPlace: + | - | + | -
bPlace: + | -
tDocu: N. Seidle

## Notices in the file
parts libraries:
SparkFun-Aesthetics: Licensing: Creative Commons ShareAlike 4.0 International - https://creativecommons.org/licenses/by-sa/4.0
SparkFun-Aesthetics: Released under the Creative Commons Attribution Share-Alike 4.0 License
SparkFun-Aesthetics: https://creativecommons.org/licenses/by-sa/4.0
